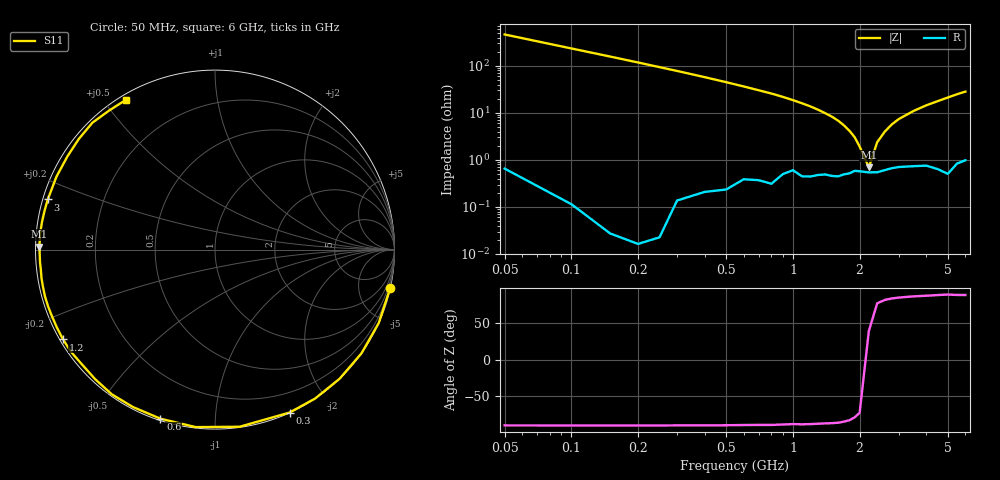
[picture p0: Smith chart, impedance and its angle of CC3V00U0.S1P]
! Infineon Technologies  Discrete & RF Semiconductors
! BBY57-02W
! Si Tuning Diode in SCD-80
! VR = 3 V
! S-Parameters:  June  2000
# GHz  S  MA  R  50
!  f  S11
! GHz  MAG  ANG
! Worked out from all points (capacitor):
!   34 points, 50 MHz to 6 GHz, reference 50 ohm
!   read as one part to ground: C = 6.78 pF near 50 MHz
!   lowest |Z| = 697 mohm at 2.2 GHz (marker M1)
!   series resonance near 2.162 GHz, so ESL is about 800 pH
!   S11 on the Smith chart (normalised r, x): 50 MHz: 0.01, -9.28; 300 MHz: 0.00, -1.56; 600 MHz: 0.01, -0.73; 1.2 GHz: 0.01, -0.27; 3 GHz: 0.01, +0.15; 6 GHz: 0.02, +0.57
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0.05  0.9997 -12.3
0.1  0.9998 -24.1
0.15  0.9999 -35.3
0.2  0.9999 -46.0
0.25  0.9998 -56.1
0.3  0.9984 -65.4
0.4  0.9964 -82.1
0.5  0.9948 -96.2
0.6  0.9899 -107.9
0.7  0.9892 -117.6
0.8  0.9902 -125.5
0.9  0.9834 -132.7
1  0.979 -139.1
1.1  0.9839 -144.6
1.2  0.9836 -149.4
1.4  0.9813 -157.8
1.6  0.9826 -164.5
1.8  0.9796 -170.6
2.2  0.9785 179.0
2.4  0.9784 174.7
2.6  0.9761 170.9
3  0.9727 163.3
3.5  0.9723 155.3
4  0.9725 147.7
4.5  0.9776 140.9
5  0.983 134.0
5.5  0.9735 127.1
6  0.9707 120.9
